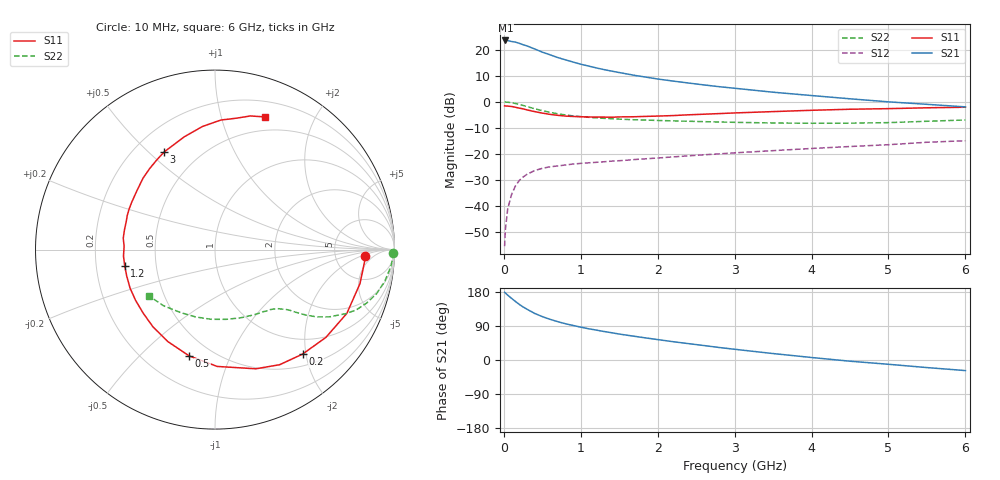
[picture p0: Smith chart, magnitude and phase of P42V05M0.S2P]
! SIEMENS Small Signal Semiconductors
! BFP182
! Si NPN RF Bipolar Junction Transistor in SOT143
! VCE = 2 V  IC = 5 mA
! Common Emitter S-Parameters:  March  1996
# GHz  S  MA  R  50
!  f  S11  S21  S12  S22
! GHz  MAG  ANG  MAG  ANG  MAG  ANG  MAG  ANG
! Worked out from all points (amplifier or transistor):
!   36 points, 10 MHz to 6 GHz, reference 50 ohm
!   highest |S21| = 23.6 dB at 20 MHz (marker M1)
!   |S21| within 3 dB of that: start of sweep to 377.8 MHz
!   unconditionally stable (mu >= 1): 1.554 GHz to 5.495 GHz
!   at 250 MHz: K = 0.22, MSG = 25.4 dB, |S12| = -28.8 dB
!   at 1.4 GHz: K = 0.94, MSG = 17.3 dB, |S12| = -22.7 dB
!   at 6 GHz: K = 0.95, MSG = 6.5 dB, |S12| = -14.9 dB
!   lowest NFmin = 1.20 dB at 450 MHz
!   S11 on the Smith chart (normalised r, x): 10 MHz: 11, -3; 200 MHz: 0.70, -1.94; 500 MHz: 0.38, -0.71; 1.2 GHz: 0.33, -0.08; 3 GHz: 0.32, +0.56; 6 GHz: 0.35, +1.38
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0.01  0.8378 -2.5  14.87 178.5  0.0017 84.6  0.9905 -1.0
0.02  0.8351 -5.2  15.11 176.9  0.0035 79.8  0.9921 -2.1
0.05  0.8297 -13.2  15.01 171.1  0.0088 84.8  0.9849 -5.4
0.1  0.8161 -25.8  14.42 162.8  0.0166 75.5  0.9627 -10.5
0.15  0.788 -38.4  14.04 154.5  0.0242 69.4  0.933 -15.3
0.2  0.7597 -50.0  13.33 146.9  0.0309 64.8  0.895 -19.5
0.25  0.7355 -60.7  12.5 140.1  0.0361 59.4  0.8559 -23.1
0.3  0.7019 -71.1  11.88 134.1  0.0406 55.7  0.813 -26.0
0.4  0.6511 -88.9  10.38 123.0  0.048 48.7  0.7387 -30.5
0.5  0.6093 -103.7  9.015 114.5  0.0531 43.6  0.679 -33.5
0.6  0.576 -117.1  8.022 107.4  0.0567 40.7  0.6303 -35.5
0.7  0.5519 -128.8  7.102 101.2  0.059 38.3  0.5913 -37.0
0.8  0.5344 -138.4  6.425 95.7  0.0614 36.5  0.5615 -38.1
1.1  0.5134 -163.3  4.879 82.5  0.0677 33.5  0.5062 -41.0
1.2  0.5111 -169.7  4.496 79.0  0.0691 32.8  0.4943 -42.0
1.7  0.5187 162.5  3.229 62.5  0.0783 32.7  0.4534 -47.6
2.2  0.5459 142.5  2.509 48.3  0.0879 32.5  0.4324 -54.8
3  0.6133 117.5  1.827 28.3  0.1052 30.8  0.4053 -69.9
3.5  0.6511 105.3  1.534 17.0  0.1159 28.7  0.3934 -81.0
4.5  0.7226 87.4  1.146 -3.2  0.1391 24.0  0.3905 -106.3
5.5  0.7701 75.2  0.898 -20.0  0.1679 18.6  0.4244 -132.5
6  0.7898 69.4  0.802 -27.9  0.1797 14.3  0.4498 -145.1
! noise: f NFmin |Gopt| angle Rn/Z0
0.45  1.2  0.27  37  0.3
0.9  1.3  0.25  75  0.23
1.8  1.9  0.21  145  0.2
